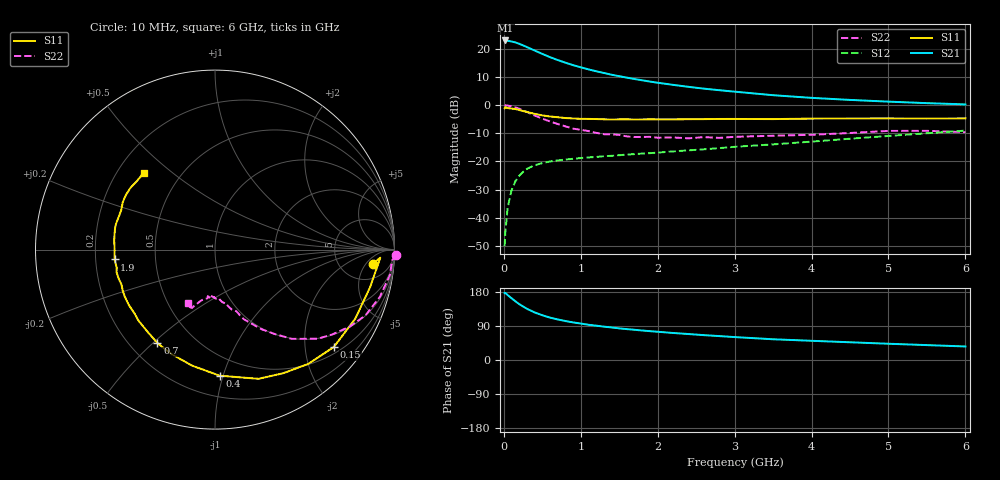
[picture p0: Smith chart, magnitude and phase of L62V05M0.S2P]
!  INFINEON TECHNOLOGIES Small Signal Semiconductors
! BFR380L3 , Si-NPN RF-Transistor in TSLP-3-1
!  Vce=2 V,  Ic=5 mA
! Common Emitter S-Parameters:  07. March 2005
#  GHz  S  MA  R  50
! f  S11  S21  S12  S22
! GHz  Mag  Ang  Mag  Ang  Mag  Ang  Mag  Ang
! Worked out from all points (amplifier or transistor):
!   36 points, 10 MHz to 6 GHz, reference 50 ohm
!   highest |S21| = 23.1 dB at 20 MHz (marker M1)
!   |S21| within 3 dB of that: start of sweep to 352.6 MHz
!   unconditionally stable (mu >= 1): 2.37 GHz to 4.747 GHz
!   at 250 MHz: K = 0.17, MSG = 22.5 dB, |S12| = -23.7 dB
!   at 1.4 GHz: K = 0.77, MSG = 14.4 dB, |S12| = -18.0 dB
!   at 6 GHz: K = 0.95, MSG = 4.7 dB, |S12| = -9.0 dB
!   S11 on the Smith chart (normalised r, x): 10 MHz: 11, -8; 150 MHz: 0.65, -2.66; 400 MHz: 0.35, -0.97; 700 MHz: 0.31, -0.52; 1.9 GHz: 0.28, -0.05; 6 GHz: 0.31, +0.40
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0.01  0.8832 -5.1  14.2 176.6  0.0031 84.9  1.012 -1.7
0.02  0.922 -2.8  14.21 176.8  0.0056 91.6  0.9885 -3.4
0.05  0.8895 -13.5  14.06 171.3  0.0152 84.9  0.9851 -8.2
0.1  0.8712 -26.2  13.61 163.0  0.0306 77.3  0.9556 -16.0
0.15  0.8561 -39.3  13.12 154.9  0.0445 70.0  0.9153 -23.6
0.2  0.8218 -50.8  12.39 147.5  0.0555 65.1  0.8651 -29.7
0.25  0.7871 -61.0  11.61 141.2  0.0652 60.0  0.8072 -35.8
0.3  0.7596 -71.4  10.82 135.2  0.0736 56.0  0.7584 -40.9
0.4  0.7029 -87.9  9.42 125.5  0.0855 50.0  0.656 -49.3
0.5  0.6592 -101.1  8.195 118.2  0.0933 46.0  0.5761 -54.7
0.6  0.6305 -112.7  7.172 111.8  0.0997 43.3  0.5149 -59.6
0.7  0.6116 -121.6  6.374 107.1  0.1039 41.8  0.4627 -63.5
0.9  0.5817 -137.1  5.166 99.2  0.1112 40.1  0.3836 -69.7
1.1  0.5708 -147.3  4.344 93.0  0.1178 40.4  0.3467 -74.4
1.4  0.5561 -159.5  3.492 85.9  0.1257 41.7  0.3039 -79.5
1.9  0.5622 -174.4  2.634 76.1  0.1403 45.2  0.2735 -89.3
2.2  0.5597 179.0  2.305 71.3  0.1507 47.5  0.2672 -91.0
2.6  0.5659 171.9  1.972 65.6  0.1641 50.7  0.2707 -95.4
3.5  0.5665 157.5  1.508 54.7  0.2009 55.1  0.2862 -103.6
4.5  0.5821 148.9  1.243 46.8  0.2534 59.1  0.3204 -108.7
5.5  0.5789 138.7  1.089 39.3  0.3169 59.5  0.35 -113.7
6  0.5839 132.8  1.034 35.7  0.3531 58.4  0.3314 -116.7
